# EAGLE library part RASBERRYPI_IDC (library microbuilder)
Rasberry PI IDC Header
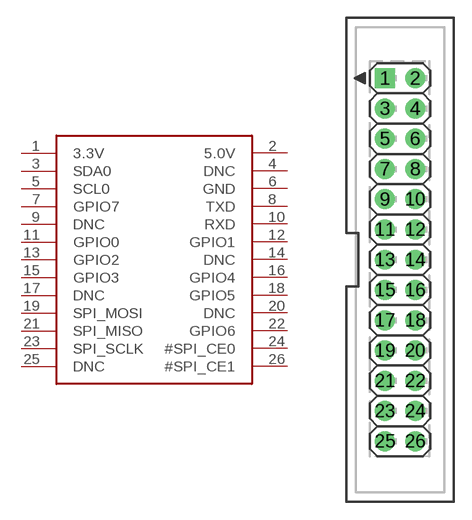
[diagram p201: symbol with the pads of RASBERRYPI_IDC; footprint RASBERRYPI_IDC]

Designator prefix JP

## RASBERRYPI_IDC  [RASBERRYPI_IDC]
1  3.3V  sup
2  5.0V  sup
3  SDA0
4  DNC  nc
5  SCL0  out
6  GND  sup
7  GPIO7
8  TXD  out
9  DNC  nc
10  RXD  in
11  GPIO0
12  GPIO1
13  GPIO2
14  DNC  nc
15  GPIO3
16  GPIO4
17  DNC  nc
18  GPIO5
19  SPI_MOSI  out
20  DNC  nc
21  SPI_MISO  in
22  GPIO6
23  SPI_SCLK  out
24  #SPI_CE0  out
25  DNC  nc
26  #SPI_CE1  out

## Footprint RASBERRYPI_IDC (pad centres in mm)
drill 1 pad 1.676 square: 1 -1.27,15.24
drill 1 pad 1.676: 2 1.27,15.24; 3 -1.27,12.7; 4 1.27,12.7; 5 -1.27,10.16; 6 1.27,10.16; 7 -1.27,7.62; 8 1.27,7.62; 9 -1.27,5.08; 10 1.27,5.08; 11 -1.27,2.54; 12 1.27,2.54; 13 -1.27,0; 14 1.27,0; 15 -1.27,-2.54; 16 1.27,-2.54; 17 -1.27,-5.08; 18 1.27,-5.08; 19 -1.27,-7.62; 20 1.27,-7.62; 21 -1.27,-10.16; 22 1.27,-10.16; 23 -1.27,-12.7; 24 1.27,-12.7; 25 -1.27,-15.24; 26 1.27,-15.24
